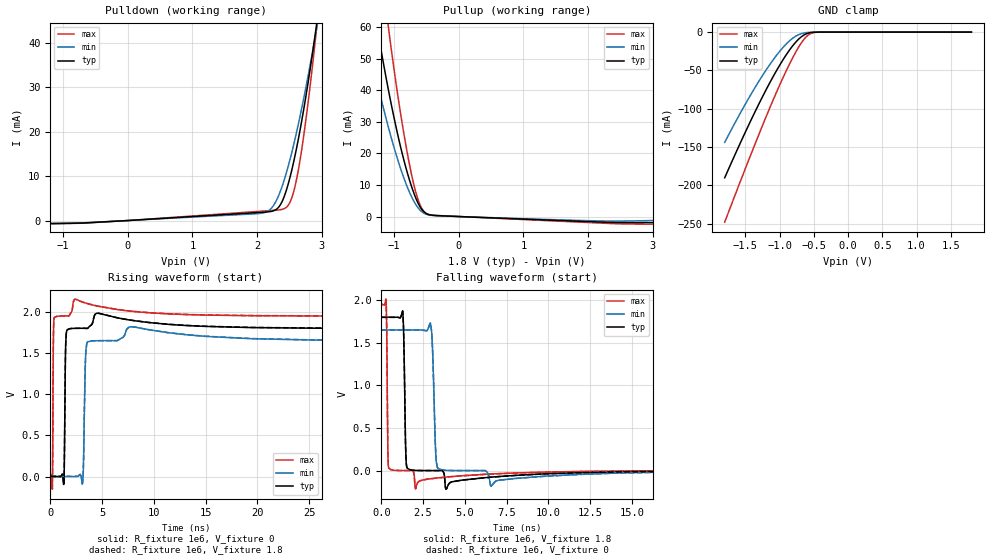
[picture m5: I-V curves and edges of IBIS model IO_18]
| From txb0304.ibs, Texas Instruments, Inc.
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[Model]   IO_18
Model_type  3-state
Enable   Active-High
Vref =   0
Rref =   1e6
Cref =   100p
Vmeas =   0.9
| variable   typ   min   max
C_comp   3.79pF   3.49pF   3.98pF
| C_pullup   4.07pF   3.75pF   4.25pF
| C_pulldown   4.06pF   3.75pF   4.24pF
| C_tri-state   3.79pF   3.49pF   3.98pF
[Temperature Range]   40   100   -40
| Ambient temperature   25   85   -40
[Voltage range]   1.8   1.65   1.95
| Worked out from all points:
|   slope of the pulldown table from 0 to 0.27 V, typ, clamps not added: 1.11 kohm
|   slope of the pullup table from 0 to 0.27 V, typ, clamps not added: 1.21 kohm
|   GND clamp passes 1 mA (typ) near -0.56 V on its own axis
|   rising waveform, R_fixture 1e6, V_fixture 0: 20-80 % time 87.8ps typ, 144ps min, 52.7ps max; typ from 0 V to 1.8 V
|   falling waveform, R_fixture 1e6, V_fixture 1.8: 20-80 % time 88ps typ, 145ps min, 55.7ps max; typ from 1.8 V to 0.002 V
|   rising waveform, R_fixture 1e6, V_fixture 1.8: 20-80 % time 87.9ps typ, 144ps min, 52.8ps max; typ from 0.002 V to 1.8 V
|   falling waveform, R_fixture 1e6, V_fixture 0: 20-80 % time 88.1ps typ, 146ps min, 55.8ps max; typ from 1.8 V to 0 V
[GND Clamp]
| IO_18
|   Voltage   I(typ)   I(min)   I(max)
-1.8V     -190.1mA   -143.9mA   -248mA
-1.585V   -147.2mA   -107.8mA   -197.9mA
-1.39V    -110mA     -77.2mA    -153.3mA
-1.215V   -78.52mA   -52.06mA   -114.6mA
-1.055V   -52.01mA   -31.68mA   -80.7mA
-910mV    -30.68mA   -16.27mA   -52.03mA
-785mV    -15.38mA   -6.585mA   -29.67mA
-675mV    -5.707mA   -1.924mA   -13.21mA
-585mV    -1.52mA    -502.6uA   -4.193mA
-515mV    -365.4uA   -143.1uA   -1.022mA
-410mV    -26.79uA   -12.71uA   -53.57uA
1.8V      536.5pA    69.43nA    35.18pA
[Pulldown]
| IO_18
|   Voltage   I(typ)   I(min)   I(max)
-1.8V     -774.1uA   -745uA     -797.5uA
-700mV    -565.3uA   -527uA     -601.8uA
2.075V    1.853mA    1.654mA    2.111mA
2.26V     2.219mA    3.503mA    2.299mA
2.36V     3.53mA     6.561mA    2.437mA
2.43V     5.792mA    9.58mA     2.737mA
2.535V    11.2mA     15.17mA    5.014mA
2.64V     18.39mA    21.76mA    11.44mA
2.755V    27.89mA    29.92mA    22.59mA
2.91V     42.92mA    42.2mA     41.72mA
2.925V    44.49mA    43.46mA    43.78mA
3.6V      131.3mA    108.3mA    163.7mA
[Pullup]
| IO_18
|   Voltage   I(typ)   I(min)   I(max)
-1.8V     132.1mA    93.14mA    198.1mA
-1.445V   82.9mA     58.43mA    124mA
-1.26V    59.37mA    42.13mA    88.89mA
-1.09V    40.11mA    28.25mA    59.94mA
-900mV    21.92mA    15.11mA    32.41mA
-765mV    11.63mA    7.743mA    16.57mA
-650mV    5.082mA    3.304mA    6.558mA
-590mV    2.739mA    1.836mA    3.24mA
-535mV    1.398mA    1.009mA    1.494mA
-360mV    317.2uA    277.5uA    353uA
2.095V    -1.673mA   -1.358mA   -1.979mA
3.6V      -1.802mA   -955.8uA   -2.439mA
[Ramp]
| IO_18
| variable   typ   min   max
dV/dt_r   1.24/1.28E-10   1.15/2.02E-10   1.39/7.25E-11
dV/dt_f   1.25/1.15E-10   1.14/1.82E-10   1.34/6.77E-11
R_load = 1e6
[Rising Waveform]
| IO_18
R_fixture =   1e6
C_fixture =   0
L_fixture =   0
V_fixture =   0
V_fixture_min = 0
V_fixture_max = 0
|   Time   V(typ)   V(min)   V(max)
0s        427.8nV    2.16uV     53.7nV
197ps     419.5nV    2.16uV     -153.4mV
365ps     5.551uV    2.16uV     1.921V
1.325ns   -79.53mV   2.459uV    1.95V
1.541ns   1.73V      6.849uV    1.95V
2.405ns   1.799V     89.41uV    2.155V
3.125ns   1.8V       -70.43mV   2.118V
3.557ns   1.798V     1.626V     2.101V
7.781ns   1.898V     1.818V     2.007V
117.2ns   1.798V     1.648V     1.948V
[Falling Waveform]
| IO_18
R_fixture =   1e6
C_fixture =   0
L_fixture =   0
V_fixture =   1.8
V_fixture_min = 1.65
V_fixture_max = 1.95
|   Time   V(typ)   V(min)   V(max)
0s        1.8V       1.65V      1.95V
293ps     1.8V       1.65V      1.968V
437ps     1.8V       1.65V      32.77mV
1.277ns   1.874V     1.65V      425.8uV
1.493ns   84.44mV    1.65V      234.3uV
2.045ns   1.949mV    1.65V      -214mV
2.957ns   142.5uV    1.711V     -95.61mV
3.365ns   34.57uV    33.92mV    -86.38mV
6.581ns   -76.65mV   -183.7mV   -39.5mV
117.2ns   1.983mV    2.066mV    1.907mV
[Rising Waveform]
| IO_18
R_fixture =   1e6
C_fixture =   0
L_fixture =   0
V_fixture =   1.8
V_fixture_min = 1.65
V_fixture_max = 1.95
|   Time   V(typ)   V(min)   V(max)
0s        1.98mV     2.064mV    1.901mV
197ps     1.98mV     2.064mV    -151.5mV
365ps     1.985mV    2.064mV    1.921V
1.325ns   -77.58mV   2.065mV    1.95V
1.541ns   1.731V     2.069mV    1.95V
2.405ns   1.799V     2.151mV    2.155V
3.125ns   1.8V       -68.37mV   2.118V
3.557ns   1.798V     1.626V     2.101V
7.781ns   1.899V     1.819V     2.009V
117.2ns   1.8V       1.65V      1.95V
[Falling Waveform]
| IO_18
R_fixture =   1e6
C_fixture =   0
L_fixture =   0
V_fixture =   0
V_fixture_min = 0
V_fixture_max = 0
|   Time   V(typ)   V(min)   V(max)
0s        1.798V     1.648V     1.948V
293ps     1.798V     1.648V     1.966V
437ps     1.798V     1.648V     32.73mV
1.277ns   1.872V     1.648V     420.8uV
1.493ns   84.11mV    1.648V     229.4uV
2.045ns   1.94mV     1.648V     -214mV
2.957ns   136.4uV    1.709V     -95.95mV
3.365ns   28.59uV    33.85mV    -86.86mV
6.581ns   -77.51mV   -183.8mV   -40.74mV
117.2ns   3.387uV    4.721uV    5.984uV
